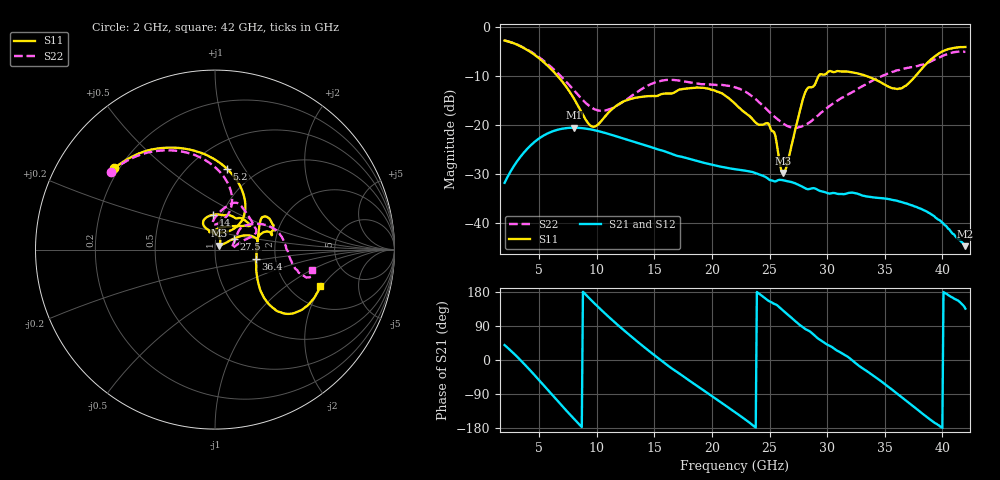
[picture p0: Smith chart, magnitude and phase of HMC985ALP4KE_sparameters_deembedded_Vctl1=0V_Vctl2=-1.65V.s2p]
!s2p File: Measurements: S11, S21, S12, S22
# GHz S dB R 50.0
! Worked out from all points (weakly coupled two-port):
!   401 points, 2 GHz to 42 GHz, reference 50 ohm
!   highest |S21| = -20.55 dB at 8 GHz (marker M1); lowest = -44.6 dB at 42 GHz (marker M2)
!   lowest |S11| = -29.8 dB at 26.2 GHz (marker M3), VSWR 1.07, Z = 52.4 + j2.33 ohm
!   |S11| at or under -10 dB: 6.581 GHz to 29.27 GHz (22.69 GHz wide, 127 % of centre); 33.36 GHz to 37.69 GHz (4.336 GHz wide, 12.2 % of centre)
!   |S22| runs from -20.6 to -2.8 dB; largest |S21 - S12| = 0.00016
!   S11 on the Smith chart (normalised r, x): 2 GHz: 0.18, +0.34; 5.2 GHz: 0.74, +0.84; 14 GHz: 0.91, +0.37; 27.5 GHz: 1.22, +0.15; 36.4 GHz: 1.58, -0.18; 42 GHz: 2.90, -1.91
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2  -2.83 141.2  -31.74 39.3  -31.74 39.3  -2.82 143.1
3.5  -4.15 113.7  -26.09 -4.1  -26.10 -4.1  -4.10 117.6
5.2  -6.84 81.5  -22.41 -60.2  -22.41 -60.2  -6.60 91.2
8  -14.55 46.5  -20.55 -154.5  -20.55 -154.6  -12.89 69.0
8.7  -17.53 52.0  -20.63 -176.9  -20.63 -176.9  -14.71 72.3
9.8  -20.34 87.7  -21.05 149.4  -21.05 149.4  -16.80 84.5
11.9  -15.77 114.0  -22.44 90.4  -22.44 90.4  -15.88 93.5
14  -14.25 92.5  -23.96 36.9  -23.97 36.8  -12.56 77.8
15.4  -13.94 73.0  -25.01 3.5  -25.01 3.5  -11.11 68.9
19.3  -12.46 34.5  -27.67 -80.8  -27.67 -80.8  -11.70 39.2
22  -15.65 52.3  -28.97 -137.4  -28.97 -137.5  -12.33 21.4
25  -20.13 98.2  -31.15 154.6  -31.15 154.5  -17.41 14.1
26.2  -29.76 43.0  -31.24 129.7  -31.23 129.7  -19.73 6.9
27.5  -18.37 30.0  -32.14 95.7  -32.14 95.5  -20.47 7.1
28.1  -13.34 20.8  -32.85 81.8  -32.84 82.0  -20.00 12.7
28.7  -12.30 12.9  -32.87 70.5  -32.87 70.6  -19.05 19.6
31  -9.07 23.3  -34.02 22.5  -34.02 22.3  -14.87 39.5
33.3  -9.95 34.3  -34.46 -26.3  -34.48 -26.4  -11.83 33.5
35.4  -12.27 12.2  -35.08 -72.8  -35.09 -72.8  -9.45 21.7
36.4  -12.58 -12.9  -35.62 -96.5  -35.63 -96.6  -8.68 14.8
39.5  -5.81 -43.3  -38.95 -168.4  -38.94 -168.8  -6.50 -14.1
42  -4.14 -19.0  -44.62 135.5  -44.63 135.9  -5.12 -12.1
